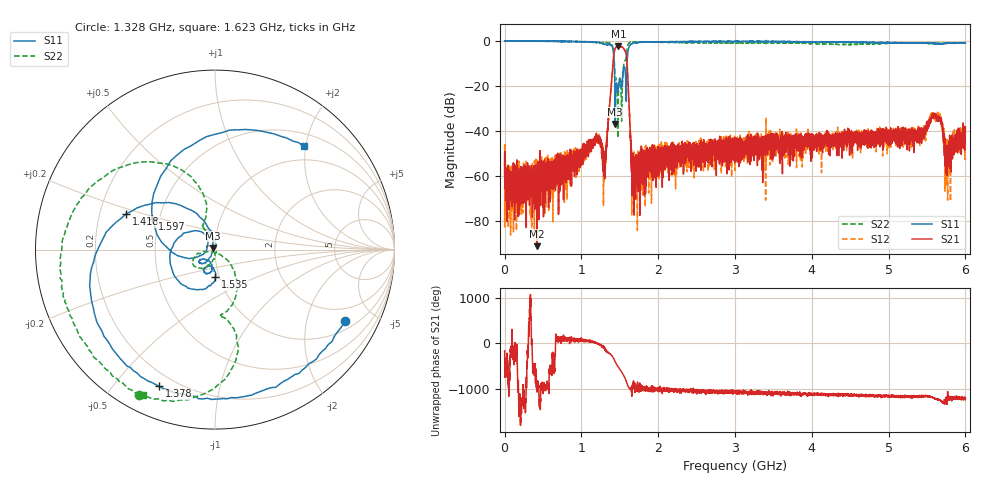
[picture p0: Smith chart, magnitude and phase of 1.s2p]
#  HZ  S  MA  R  50.00
! Rohde & Schwarz Vector Network Analyzer
! Rohde-Schwarz,ZNL6-2Port,1323001206101378,1.50.1.34-21.10.1.104
! Created: UTC 3/8/2024, 2:15:00 AM
! freq[Hz]  mag:S11  ang:S11  mag:S21  ang:S21  mag:S12  ang:S12  mag:S22  ang:S22
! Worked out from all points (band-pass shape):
!   6000 points, 5 kHz to 6 GHz, reference 50 ohm
!   highest |S21| = -2.43 dB at 1.481 GHz (marker M1); lowest = -91.3 dB at 423.1 MHz (marker M2)
!   |S21| within 3 dB of the highest: 1.425 GHz to 1.58 GHz (154.7 MHz wide, 10.3 % of centre)
!   lowest |S11| = -37.0 dB at 1.44 GHz (marker M3), VSWR 1.03, Z = 48.9 + j0.862 ohm
!   |S11| at or under -10 dB: 1.427 GHz to 1.595 GHz (167.7 MHz wide, 11.1 % of centre)
!   |S22| runs from -43.2 to 0.2 dB; largest |S21 - S12| = 0.024
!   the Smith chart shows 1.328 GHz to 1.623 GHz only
!   S11 on the Smith chart (normalised r, x): 1.328 GHz: 1.35, -3.38; 1.378 GHz: 0.14, -0.66; 1.418 GHz: 0.31, +0.17; 1.535 GHz: 0.96, -0.30; 1.597 GHz: 0.46, +0.19; 1.623 GHz: 0.72, +1.96
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5000  1.002 -0.6  0.002466 -161.3  0.004938 49.7  1.013 -0.4
7.801794e7  1.001 -13.4  0.0005418 -86.0  4.794e-05 3.4  0.9955 -18.1
4.230752e8  0.9851 -70.9  2.71e-05 14.2  0.0008625 165.8  0.9956 -92.9
1.000171e9  0.9631 -145.0  0.003045 54.8  0.003618 67.1  0.96 148.5
1.144195e9  0.9558 178.7  0.004439 31.2  0.006504 27.8  0.9306 84.2
1.225208e9  0.9254 132.9  0.006724 -5.0  0.005829 -13.1  0.9117 6.8
1.274216e9  0.8708 72.1  0.004113 -50.4  0.003695 -56.1  0.9062 -56.1
1.328225e9  0.8253 -28.9  0.00455 179.5  0.007341 -171.3  0.9158 -117.4
1.378234e9  0.8219 -112.2  0.0619 120.8  0.06402 121.9  0.869 -170.8
1.41824e9  0.5343 158.1  0.4206 36.3  0.4104 36.8  0.575 123.0
1.440244e9  0.01416 141.5  0.6856 -43.7  0.6843 -44.1  0.1659 110.6
1.481251e9  0.0863 -102.4  0.756 -158.8  0.7526 -159.3  0.06471 -102.1
1.53526e9  0.1532 -89.0  0.7209 62.8  0.7178 62.4  0.1292 -44.3
1.59727e9  0.3907 153.7  0.2608 -176.0  0.2612 -177.0  0.7111 -84.7
1.623274e9  0.758 49.3  0.02891 103.6  0.02905 102.1  0.9053 -116.4
1.680284e9  0.9001 -25.7  0.00161 -140.5  0.001093 72.9  0.9428 -147.9
2.000337e9  0.9441 -94.9  0.003181 62.6  0.003341 77.4  0.9381 153.1
3.000503e9  0.9692 -121.6  0.003728 44.3  0.005185 36.1  0.911 76.8
4.000668e9  0.9572 -125.2  0.005241 -17.3  0.004166 -25.4  0.8722 19.4
5.000834e9  0.9169 -125.7  0.008672 -67.1  0.006538 -89.4  0.8892 -30.6
5.770962e9  0.8922 -120.7  0.003862 -111.9  0.003022 -158.8  0.8819 -69.6
6e9  0.8957 -122.5  0.01212 -131.6  0.005246 -115.4  0.9132 -81.3
